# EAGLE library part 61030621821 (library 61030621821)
WURTH ELEKTRONIK - 61030621821 - Board-To-Board Connector, 2.54 mm, 6 Contacts, Receptacle, WR-PHD Series, Surface Mount, 2 Rows Source: Datasheet
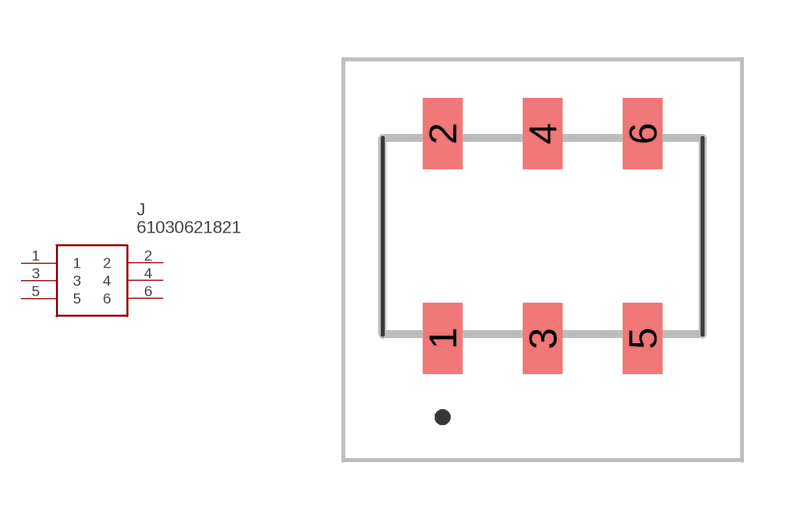
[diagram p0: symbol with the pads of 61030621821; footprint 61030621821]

Designator prefix J

## 61030621821 (Description: WURTH ELEKTRONIK - 61030621821 - Board-To-Board Connector, 2.54 mm, 6 Contacts, Receptacle, WR-PHD Series, Surface Mount, 2 Rows; Height: 7.75mm; Manufacturer_Name: Wurth Elektronik; Manufacturer_Part_Number: 61030621821; Mouser_Part_Number: 710-61030621821; Mouser_Price-Stock: https://www.mouser.co.uk/ProductDetail/Wurth-Elektronik/61030621821?qs=Cb2nCFKsA8prWiqa1E1TsA%3D%3D)  [61030621821]
1  1
2  2
3  3
4  4
5  5
6  6

## Footprint 61030621821 (pad centres in mm)
61030621821-1
smd 1 x 1.8: 1 -2.54,-2.6; 2 -2.54,2.6; 3 0,-2.6; 4 0,2.6; 5 2.54,-2.6; 6 2.54,2.6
